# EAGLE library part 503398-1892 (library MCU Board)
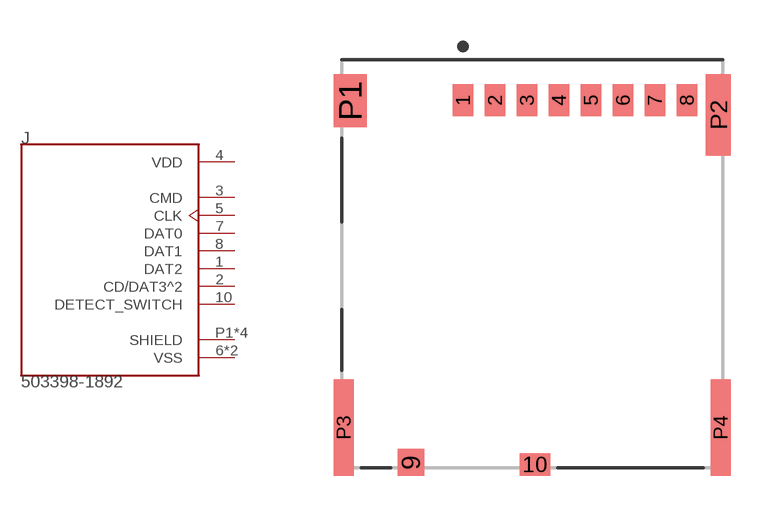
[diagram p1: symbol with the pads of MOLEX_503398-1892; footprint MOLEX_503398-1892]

Designator prefix J

## 503398-1892  [MOLEX_503398-1892]
1  DAT2  pas
2  CD/DAT3^2  pas
3  CMD  pas
4  VDD  pwr
5  CLK  pas
6  VSS  pwr
7  DAT0  pas
8  DAT1  pas
9  VSS  pwr
10  DETECT_SWITCH  pas
P1  SHIELD  pas
P2  SHIELD  pas
P3  SHIELD  pas
P4  SHIELD  pas

## Footprint MOLEX_503398-1892 (pad centres in mm)
smd 0.7 x 1.1: 1 -3.65,6.895; 2 -2.55,6.895; 3 -1.45,6.895; 4 -0.35,6.895; 5 0.75,6.895; 6 1.85,6.895; 7 2.95,6.895; 8 4.05,6.895
smd 0.9 x 0.93: 9 -5.44,-5.57
smd 1.05 x 0.78: 10 -1.175,-5.645
smd 1.14 x 1.83: P1 -7.53,6.88
smd 0.86 x 2.8: P2 5.13,6.395
smd 0.7 x 3.33: P3 -7.75,-4.37; P4 5.21,-4.37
